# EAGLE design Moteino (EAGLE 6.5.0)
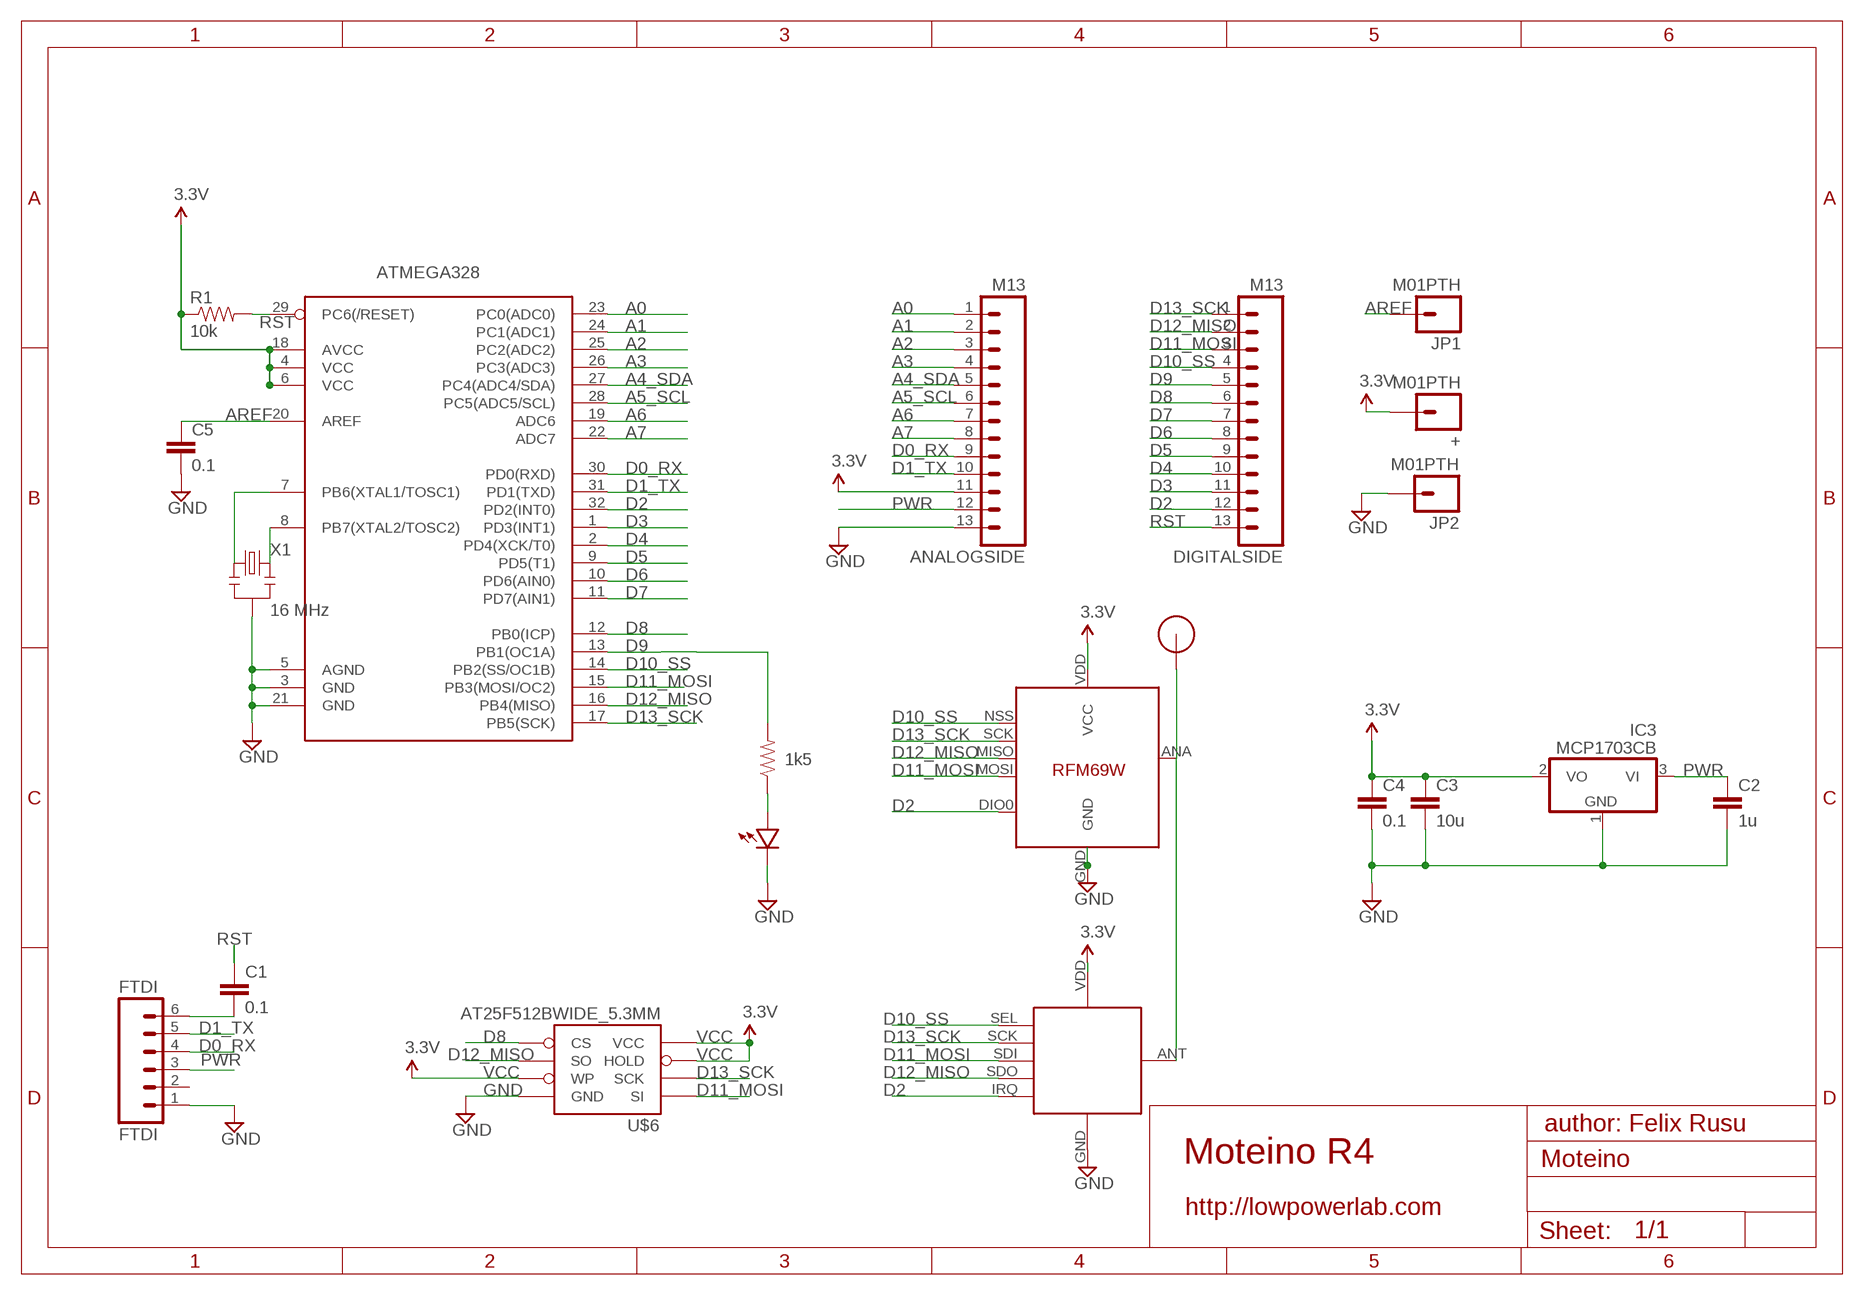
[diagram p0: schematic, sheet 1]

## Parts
+  M01PTH  [1X01]
ANALOGSIDE  M13  [1X13]
ATMEGA328  ATMega-328  ATMEGA168/328TQFP32  [TQFP32-08]
C1  0.1  CAP0603-CAP  [0603-CAP]
C2  1u  CAP0603-CAP  [0603-CAP]
C3  10u  CAP0805-CAP  [0805-CAP]
C4  0.1  CAP0603-CAP  [0603-CAP]
C5  0.1  CAP0603-CAP  [0603-CAP]
DIGITALSIDE  M13  [1X13]
FTDI  FTDI  M06SIP  [1X06]
IC3  MCP1703CB  [SOT23]
JP1  M01PTH  [1X01]
JP2  M01PTH  [1X01]
R1  10k  RESISTOR0603-RES  [0603-RES]
R2  1k5  RESISTOR0603-RES  [0603-RES]
RFM12B  RFM12B_MINPADS  [RFM12B-MINPADS]
U$1  RFM12B_ANTENNA  [RFM12B-ANTENNA]
U$2  LED0603  [0603-LED]
U$5  RFM69  [RFM69W-MINPADS]
U$6  AT25F512BWIDE_5.3MM  [SO08WIDE]
X1  16 MHz  RESONATORSMD  [RESONATOR-SMD]

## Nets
A0: ANALOGSIDE.1 ATMEGA328.23(PC0(ADC0))
A1: ANALOGSIDE.2 ATMEGA328.24(PC1(ADC1))
A2: ANALOGSIDE.3 ATMEGA328.25(PC2(ADC2))
A3: ANALOGSIDE.4 ATMEGA328.26(PC3(ADC3))
A4_SDA: ANALOGSIDE.5 ATMEGA328.27(PC4(ADC4/SDA))
A5_SCL: ANALOGSIDE.6 ATMEGA328.28(PC5(ADC5/SCL))
A6: ANALOGSIDE.7 ATMEGA328.19(ADC6)
A7: ANALOGSIDE.8 ATMEGA328.22(ADC7)
AREF: ATMEGA328.20(AREF) C5.1 JP1.1
D0_RX: ANALOGSIDE.9 ATMEGA328.30(PD0(RXD)) FTDI.4
D1_TX: ANALOGSIDE.10 ATMEGA328.31(PD1(TXD)) FTDI.5
D2: ATMEGA328.32(PD2(INT0)) DIGITALSIDE.12 RFM12B.IRQ U$5.DIO0
D3: ATMEGA328.1(PD3(INT1)) DIGITALSIDE.11
D4: ATMEGA328.2(PD4(XCK/T0)) DIGITALSIDE.10
D5: ATMEGA328.9(PD5(T1)) DIGITALSIDE.9
D6: ATMEGA328.10(PD6(AIN0)) DIGITALSIDE.8
D7: ATMEGA328.11(PD7(AIN1)) DIGITALSIDE.7
D8: ATMEGA328.12(PB0(ICP)) DIGITALSIDE.6 U$6.1(CS)
D9: ATMEGA328.13(PB1(OC1A)) DIGITALSIDE.5 R2.2
D10_SS: ATMEGA328.14(PB2(SS/OC1B)) DIGITALSIDE.4 RFM12B.SEL U$5.NSS(SEL)
D11_MOSI: ATMEGA328.15(PB3(MOSI/OC2)) DIGITALSIDE.3 RFM12B.SDI(SDI/MOSI) U$5.MOSI U$6.5(SI)
D12_MISO: ATMEGA328.16(PB4(MISO)) DIGITALSIDE.2 RFM12B.SDO(SDO/MISO) U$5.MISO U$6.2(SO)
D13_SCK: ATMEGA328.17(PB5(SCK)) DIGITALSIDE.1 RFM12B.SCK U$5.SCK U$6.6(SCK)
GND [power]: ANALOGSIDE.13 ATMEGA328.3(GND) ATMEGA328.5(AGND) ATMEGA328.21(GND) C2.2 C3.2 C4.2 C5.2 FTDI.1 IC3.1(GND) JP2.1 RFM12B.GND U$2.MINUS U$5.GND U$6.4(GND) X1.2
N$1: ATMEGA328.7(PB6(XTAL1/TOSC1)) X1.1
N$2: R2.1 U$2.PLUS
N$3: RFM12B.ANT U$1.P$1 U$5.ANA(ANT)
N$20: C1.2 FTDI.6
N$21: ATMEGA328.8(PB7(XTAL2/TOSC2)) X1.3
PWR [power]: ANALOGSIDE.12 C2.1 FTDI.3 IC3.3(VI)
RST: ATMEGA328.29(PC6(/RESET)) C1.1 DIGITALSIDE.13 R1.2
VCC: +.1 ANALOGSIDE.11 ATMEGA328.4(VCC) ATMEGA328.6(VCC) ATMEGA328.18(AVCC) C3.1 C4.1 IC3.2(VO) R1.1 RFM12B.VDD U$5.VDD(VCC) U$6.3(WP) U$6.7(HOLD) U$6.8(VCC) ; supply symbol labelled 3.3V
Unconnected: FTDI.2

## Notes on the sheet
- author: Felix Rusu
- Moteino R4
- http://lowpowerlab.com

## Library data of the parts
+ JP1 JP2 = SparkFun-Connectors:M01: Header 1
ANALOGSIDE DIGITALSIDE = SparkFun-Connectors:M13: 13-pin single row .1" header
ATMEGA328 = LowPowerLab:ATMEGA168/328: Atmel 32-pin 8-bit micro, 16k flash.
C1-C5 = LowPowerLab:CAP: Capacitor
FTDI = SparkFun-Connectors:M06: Header 6 Standard 6-pin 0.1" header. Use with straight break away headers (SKU : PRT-00116), right angle break away headers (PRT-00553), swiss pins (PRT-00743), machine pins (PRT-00117), and female headers (PRT-00115). Molex polarized connector foot print use with SKU : PRT-08094 with associated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
IC3 = linear:MCP1703: 250 mA, 16V, Low Quiescent Current LDO Regulator Source: http://ww1.microchip.com/downloads/en/DeviceDoc/22049b.pdf
R1 R2 = LowPowerLab:RESISTOR: Resistor
RFM12B = LowPowerLab:RFM12B_MINPADS
U$1 = LowPowerLab:RFM12B_ANTENNA
U$2 = LowPowerLab:LED
U$5 = LowPowerLab:RFM69
U$6 = LowPowerLab:AT25F512B: 4-Mbit SPI flash memory
X1 = SparkFun:RESONATOR: Resonator Small SMD resonator. This is the itty bitty 10/20MHz resonators with built in caps. CSTCE10M0G55 and CSTCE20M0V53. Footprint has been reviewed closely but hasn't been tested yet.

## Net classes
1 power: width 0.381 mm, clearance 0.254 mm

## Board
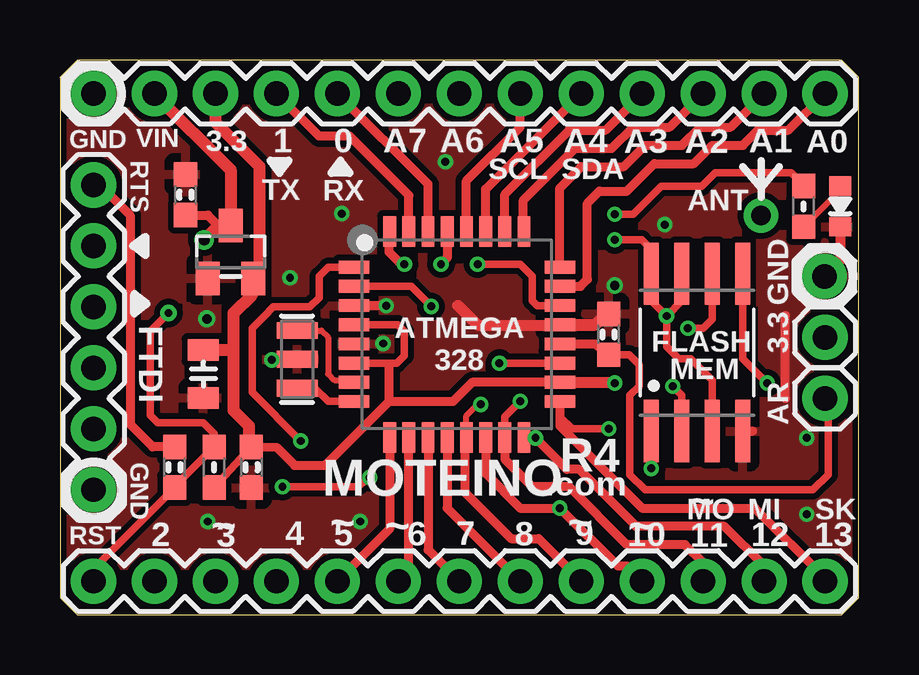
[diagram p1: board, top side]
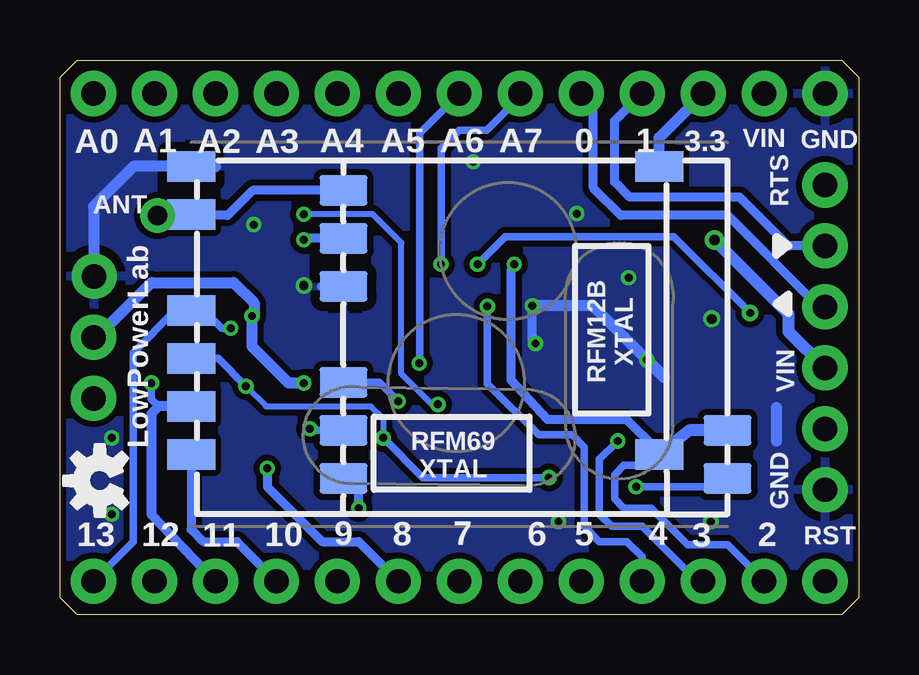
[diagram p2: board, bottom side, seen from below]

Size 33.27 x 23.11 mm. Coordinates in mm from the lower left corner, seen from the top.
Outline: 0.71,0 32.56,0 33.27,0.71 33.27,22.4 32.56,23.11 0.71,23.11 0,22.4 0,0.71 0.71,0
Copper layers (1*16): Top 0.035mm / dielectric 1.5mm / Bottom 0.035mm
Design rules "ITEADstudio_DRC *": minimum track width 6mil, minimum drill 12mil, track to track 6mil, track to pad 6mil, pad to pad 6mil, via to via 6mil, smd to smd 0mil, copper to edge 10mil, drill to drill 10mil, minimum pad ring 10mil, minimum via ring 6mil, stop-mask expansion 2mil, vias tented up to drill 100mil, thermal gap 15mil
tRestrict: area 24.3,8.9 to 29.1,12.8; area 5.8,16.9 to 6.9,18.5; area 5.2,9.7 to 6.7,10.4
bRestrict: area 27.4,17.7 to 29.2,18.7; area 21.1,13.8 to 22.9,14.9; area 21.6,12.6 to 22.1,13.2; area 20.7,12.6 to 21.2,13.2; area 20.2,12.8 to 20.7,13.5; area 20.1,13.4 to 20.6,14; area 26.5,18.9 to 27.1,19.5; area 26.5,17.9 to 27.1,18.5; area 27.5,19.1 to 28,19.8; area 27.9,18.8 to 29.1,19.6

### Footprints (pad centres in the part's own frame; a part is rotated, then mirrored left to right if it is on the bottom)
1X01 = drill 1.016 pad 1.88: 1 0,0
1X13 = drill 1.016 pad 1.88: 1 0,0; 2 2.54,0; 3 5.08,0; 4 7.62,0; 5 10.16,0; 6 12.7,0; 7 15.24,0; 8 17.78,0; 9 20.32,0; 10 22.86,0; 11 25.4,0; 12 27.94,0; 13 30.48,0
TQFP32-08 = smd 1.27 x 0.533: 1 -4.293,2.8; 2 -4.293,2; 3 -4.293,1.2; 4 -4.293,0.4; 5 -4.293,-0.4; 6 -4.293,-1.2; 7 -4.293,-2; 8 -4.293,-2.8; 17 4.293,-2.8; 18 4.293,-2; 19 4.293,-1.2; 20 4.293,-0.4; 21 4.293,0.4; 22 4.293,1.2; 23 4.293,2; 24 4.293,2.8 | smd 0.533 x 1.27: 9 -2.8,-4.293; 10 -2,-4.293; 11 -1.2,-4.293; 12 -0.4,-4.293; 13 0.4,-4.293; 14 1.2,-4.293; 15 2,-4.293; 16 2.8,-4.293; 25 2.8,4.293; 26 2,4.293; 27 1.2,4.293; 28 0.4,4.293; 29 -0.4,4.293; 30 -1.2,4.293; 31 -2,4.293; 32 -2.8,4.293
0603-CAP = smd 1.016 x 0.965: 1 -0.85,0; 2 0.85,0
0805-CAP = smd 0.902 x 1.3: 1 -1,0; 2 1,0
1X06 = drill 1.016 pad 1.88: 1 0,0; 2 2.54,0; 3 5.08,0; 4 7.62,0; 5 10.16,0; 6 12.7,0
SOT23 = smd 1 x 1.4: 1 -0.95,-1.1; 2 0.95,-1.1; 3 0,1.1
0603-RES = smd 1.016 x 0.965: 1 -0.85,0; 2 0.85,0
RFM12B-MINPADS = smd 2 x 1.27: ANT 8,-6; GND 8,-2; IRQ -8,4; SCK 8,4; SDI 8,2; SDO -8,6; SEL 8,6; VDD 8,-4
RFM12B-ANTENNA = drill 0.8 pad 1.422: P$1 0,0
0603-LED = smd 0.8 x 0.9: MINUS -0.85,0; PLUS 0.85,0
RFM69W-MINPADS = smd 2 x 1.27: ANA 8,-5; DIO0 -11.5,5; GND 8,-7; MISO 8,1; MOSI 8,3; NSS 8,5; SCK 8,-1; VDD -11.5,-7
SO08WIDE = smd 0.61 x 2.6: 1 -1.905,-3.269; 2 -0.635,-3.269; 3 0.635,-3.269; 4 1.905,-3.269; 5 1.905,3.286; 6 0.635,3.286; 7 -0.635,3.286; 8 -1.905,3.286
RESONATOR-SMD = smd 0.7 x 1.7: 1 -1.2,0; 2 0,0; 3 1.2,0

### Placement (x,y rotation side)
+  31.88,11.56 270 top
ANALOGSIDE  31.88,21.72 180 top
ATMEGA328  16.54,11.68 0 top
C1  4.78,6.15 90 top
C2  5.23,17.5 90 top
C3  5.97,10.03 270 top
C4  7.98,6.15 270 top
C5  22.86,11.68 90 top
DIGITALSIDE  31.88,1.4 180 top
FTDI  1.4,5.21 90 top
IC3  7.11,15.11 0 top
JP1  31.88,9.02 0 top
JP2  31.85,14.1 0 top
R1  6.43,6.15 90 top
R2  30.99,17.02 90 top
RFM12B  13.46,11.68 180 bottom
U$1  29.21,16.64 0 top
U$2  32.51,17.02 90 top
U$3  [OSHW-LOGO-S]  31.62,5.59 90 bottom
U$5  19.81,11.68 180 bottom
U$6  26.54,10.92 0 top
X1  9.88,10.64 270 top

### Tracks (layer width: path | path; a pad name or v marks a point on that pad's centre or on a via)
A0
  Top 0.381: ATMEGA328.23 21.68,13.68 21.97,13.97 21.97,17.14 22.48,17.65 23.62,17.65 24.77,18.8 26.42,18.8 27.18,19.56 28.45,19.56 29.08,20.19 30.35,20.19 ANALOGSIDE.1
A1
  Top 0.381: ATMEGA328.24 20.83,17.78 21.72,18.67 23.5,18.67 24.38,19.56 25.91,19.56 26.67,20.32 27.94,20.32 ANALOGSIDE.2
A2
  Top 0.381: ATMEGA328.25 19.3,15.98 19.3,17.27 21.46,19.43 22.99,19.43 23.88,20.32 25.4,20.32 ANALOGSIDE.3
A3
  Top 0.381: ATMEGA328.26 18.54,17.52 21.21,20.19 22.73,20.19 ANALOGSIDE.4
A4_SDA
  Top 0.381: ATMEGA328.27 17.73,17.73 ANALOGSIDE.5
A5_SCL
  Top 0.381: ATMEGA328.28 16.93,18.08 19.18,20.32 ANALOGSIDE.6
A6  (via drill 0.33)
  Top 0.305: ATMEGA328.19 v18.31,10.48
  Bottom 0.305: 18.29,10.41 18.29,20.07 ANALOGSIDE.7
  Bottom 0.381: 18.29,10.41 v18.31,10.48
A7  (via drill 0.33)
  Top 0.305: ATMEGA328.22 19.88,12.88 19.68,13.08 19.68,14.1 19.18,14.61 v17.4,14.61
  Bottom 0.305: v17.4,14.61 17.4,19.43 16.64,20.19 15.49,20.19 14.1,21.59 ANALOGSIDE.8
AREF
  Top 0.305: C5.1 23.71,10.83 24.13,10.41 24.13,9.53 23.75,9.14 23.75,5.84 24.38,5.21 31.37,5.21 32,5.84 32,8.89 JP1.1
  Top 0.381: ATMEGA328.20 22.28,11.28 C5.1
D0_RX
  Top 0.381: ATMEGA328.30 15.34,17.94 ANALOGSIDE.9
  Bottom 0.381: FTDI.4 1.65,12.83 5.46,16.64 9.91,16.64 11.05,17.78 11.05,21.21 ANALOGSIDE.9 11.68,21.59
D1_TX
  Top 0.381: ATMEGA328.31 14.54,17.47 12.06,19.94 10.79,19.94 ANALOGSIDE.10
  Bottom 0.381: FTDI.5 2.92,15.37 4.95,17.4 9.53,17.4 10.16,18.03 10.16,20.57 ANALOGSIDE.10
D2  (via drill 0.33)
  Top 0.381: v14.35,14.61 14.22,14.61 13.72,15.11 13.72,15.83 ATMEGA328.32
  Bottom 0.305: DIGITALSIDE.12 5.46,2.92 7.11,2.92 8.64,4.45 9.78,4.45 10.16,4.83 10.16,5.84 9.78,6.22 8.77,6.22 U$5.DIO0
  Bottom 0.381: 7.85,6.89 8.41,6.89 9.65,8.13 12.95,8.13 14.48,9.78 14.48,14.35 v14.35,14.61
  Bottom 0.406: U$5.DIO0 8.05,6.68 7.85,6.89
  Bottom 0.508: RFM12B.IRQ 7.06,7.68 U$5.DIO0
D3  (via drill 0.33)
  Top 0.305: v10.03,7.24 8,9.27 8,11.05 8,11.94 8.51,12.45 8.89,12.83 10.41,12.83 10.79,13.21 10.79,14.1 11.18,14.48 ATMEGA328.1
  Top 0.381: ATMEGA328.1
  Bottom 0.305: DIGITALSIDE.11 6.73,1.4 9.02,3.68 10.29,3.68 10.79,4.19 10.79,6.48 v10.03,7.24
D4  (via drill 0.33)
  Top 0.305: ATMEGA328.2 14.63,13.68 v15.46,12.85
  Top 0.381: 12.17,13.73 ATMEGA328.2
  Bottom 0.305: DIGITALSIDE.10 9.02,2.41 9.65,3.05 10.79,3.05 11.43,3.68 11.43,6.99 11.94,7.49 13.34,7.49 15.46,9.62 v15.46,12.85
D5
  Top 0.381: ATMEGA328.9 13.73,3.58 DIGITALSIDE.9
D6
  Top 0.381: DIGITALSIDE.8 14.54,1.83 ATMEGA328.10
D7
  Top 0.381: ATMEGA328.11 15.34,2.7 DIGITALSIDE.7
D8  (via drill 0.33)
  Top 0.305: v24.64,6.1 24.62,7.75 U$6.1
  Top 0.381: ATMEGA328.12 16.14,4.44 DIGITALSIDE.6
  Bottom 0.381: v24.64,6.1 24.64,5.33 22.35,3.05 20.83,3.05 DIGITALSIDE.6
D9  (via drill 0.33)
  Top 0.254: ATMEGA328.13 16.93,8.3 17.4,8.76 v17.53,8.76
  Top 0.305: R2.2 30.77,18.12 30.48,18.41 27.3,18.41 26.75,17.86 25.04,17.86 23.88,16.69 v23.11,16.69
  Top 0.381: ATMEGA328.13 16.89,7.31 16.89,5.08 18.8,3.17 19.94,3.17 DIGITALSIDE.5
  Bottom 0.254: v17.53,8.76 17.78,8.76 19.05,10.03 19.05,15.49 20.24,16.69 v23.11,16.69
D10_SS  (via drill 0.33)
  Top 0.381: ATMEGA328.14 17.73,5.89 19.18,4.45 v20.83,4.45 23.24,2.03 23.62,2.03 DIGITALSIDE.4
  Bottom 0.254: 20.83,5.43 RFM12B.SEL
  Bottom 0.381: v20.83,4.45 20.83,5.43 | U$5.NSS 27.81,3.56 27.3,3.05 25.91,3.05 DIGITALSIDE.4
D11_MOSI  (via drill 0.33)
  Top 0.305: v29.46,9.65 28.45,10.67 U$6.5 | ATMEGA328.15 18.54,8.25 v19.18,8.89
  Top 0.381: ATMEGA328.15 18.54,6.48 19.68,5.33 21.21,5.33 23.62,2.92 26.04,2.92 26.8,2.16 DIGITALSIDE.3
  Bottom 0.305: v29.46,9.65 29.46,8.99 29.16,8.68 | v19.18,8.89 19.97,9.68 RFM12B.SDI
  Bottom 0.381: DIGITALSIDE.3 29.46,4.19
  Bottom 0.406: U$5.MOSI 29.16,8.68 29.46,8.38 29.46,4.19
D12_MISO  (via drill 0.33)
  Top 0.305: v25.53,9.53 25.91,9.14 25.91,8.51 U$6.2 | v9.27,5.33 12.39,5.33 v12.9,5.71
  Top 0.381: ATMEGA328.16 19.91,7.39 v19.81,7.37 21.12,6.06 21.63,6.06 24,3.68 27.69,3.68 29.34,2.03 DIGITALSIDE.2
  Bottom 0.254: v25.53,9.53 24.69,8.69 20.32,8.69 19.81,8.18 v19.81,7.37
  Bottom 0.305: U$5.MISO 26.69,10.68 v25.53,9.53 25.84,9.84 | v19.81,7.37 18.16,5.71 v12.9,5.71 | v9.27,5.33 5.81,5.33 RFM12B.SDO
D13_SCK  (via drill 0.33)
  Top 0.305: v26.16,11.94 26.8,11.94 27.18,12.32 U$6.6 | v22.86,7.75 21.34,7.75 20.83,8.26
  Top 0.381: DIGITALSIDE.1 31.88,1.52 28.96,4.45 24.25,4.45 20.83,7.87 20.83,8.26 ATMEGA328.17
  Bottom 0.305: RFM12B.SCK 22.8,7.68 v22.86,7.75 | DIGITALSIDE.1 30.23,3.05 30.23,10.92 28.46,12.68 U$5.SCK 27.8,12.7 27.3,12.7 26.54,11.94 v26.16,11.94
GND  (via drill 0.33, 0.38, 0.41)
  Top 0.381: 20.94,12.06 ATMEGA328.21 | v13.59,12.88 ATMEGA328.3 | 16.53,12.88 16.59,12.88 | U$6.4 28.86,7.65 | 30.23,9.02 30.23,12.47 | v8.82,10.62 X1.2
  Top 0.406: U$2.MINUS 32.51,14.76 JP2.1
  Top 0.457: 20.94,12.06 17.4,12.06 16.59,12.88
  Top 0.508: ATMEGA328.21 22.28,12.08 C5.2 22.99,12.41
  Bottom 0.381: 13.59,12.81 v13.59,12.88 13.59,11.3 v13.46,11.3 | RFM12B.GND 22.38,13.68
  Bottom 0.457: 31.88,14.12 JP2.1 31.88,14.12 | 26.81,18.68 30.21,18.68 31.88,17.02 31.88,14.12 | v8.82,10.62 11.08,12.88 v13.59,12.88 | 3.43,8.64 3.43,7.24
  Bottom 0.508: U$5.GND 26.81,18.68 | 8.11,9.91 v8.82,10.62
  other vias: 6.12,12.32 23.11,13.72 6.15,3.89 12.5,3.89 9.58,14.05 11.74,16.71 16.06,18.87 25.2,16.26 31.11,7.37 31.11,4.19
  pour Bottom: -0.64,24 -0.64,-0.76 34.04,-0.76 34.04,24
  pour Top: -0.64,24 -0.64,-0.76 34.04,-0.76 34.04,24
N$1
  Top 0.254: X1.1 10.89,11.84 11.18,11.56 11.18,10.03 11.43,9.78 12.15,9.78 ATMEGA328.7
N$2
  Top 0.254: R2.1 32.38,17.57 U$2.PLUS
N$3
  Bottom 0.381: U$1.P$1 28.5,16.68 U$5.ANA 27.51,16.64 26.29,16.64 25.24,17.68 RFM12B.ANT
N$20
  Top 0.381: C1.2 3.86,7 2.92,7.94 2.92,16.64 1.65,17.91 FTDI.6
N$21
  Top 0.254: ATMEGA328.8
  Top 0.305: X1.3 10.62,9.44 11.18,8.89 ATMEGA328.8
PWR  (via drill 0.46 pad 0.81)
  Top 0.381: C2.1 6.17,16.65 6.6,16.21
  Top 0.508: ANALOGSIDE.12 7.11,18.54 IC3.3 6.6,16.21 v6,15.61
  Bottom 0.508: FTDI.3 2.92,11.81 2.92,12.45 2.92,12.53 v6,15.61
RST  (via drill 0.33, 0.33 pad 0.69)
  Top 0.305: DIGITALSIDE.13 1.4,1.92 C1.1 4.78,5.35 R1.2 6.43,7.54 5.97,8 4.06,8 3.76,8.31 3.76,11.81 v4.52,12.57
  Top 0.381: ATMEGA328.29 16.14,14.87 v15.88,14.61
  Bottom 0.305: v15.88,14.61 14.73,15.75 7.7,15.75 v4.52,12.57
VCC  (via drill 0.33)
  Top 0.305: ATMEGA328.4 14.08,12.08 14.35,11.81 14.35,10.79 14.03,10.48 13.84,10.48 | ATMEGA328.6 13.84,10.48 | v25.27,12.45 24.64,13.08 U$6.8 | v25.27,12.45 25.91,13.08 U$6.7 | v25.27,12.45 25.27,11.18 25.78,10.67 26.29,10.67 27.18,9.78 U$6.3 | v23.11,15.62 24.24,15.62 24.64,15.22 | 13.72,10.36 13.84,10.48 | R1.1 6.43,5.32 C4.1
  Top 0.381: 24.64,15.22 U$6.8 | ATMEGA328.18 17.18,9.68 16.38,8.89 13.72,8.89 | 13.72,8.89 13.72,10.36 | C4.1 9.03,6.97 9.78,6.22 11.05,6.22 13.72,8.89
  Top 0.457: ATMEGA328.18 23.21,9.68 v23.11,9.65
  Top 0.508: 7.87,7.07 C4.1 7.87,7.07 | C3.1 6.24,11.03 7.22,11.03 7.24,11.05 | 7.87,7.07 7.87,7.87 7.24,8.51 7.24,11.05 | 7.24,11.05 7.24,12.57 8,13.34 8,13.95 IC3.2 | IC3.2 8.23,13.84 | ANALOGSIDE.11 6.48,20.52 U$5.VDD 8.31,14.26 IC3.2
  Top 0.635: 8.23,13.73 8.23,13.84
  Bottom 0.381: RFM12B.VDD 23.18,15.68 v23.11,15.62
  Bottom 0.457: +.1 31.75,11.56 29.46,13.84 26.04,13.84 25.18,12.99 25.18,12.54 v25.27,12.45 25.27,11.18 23.75,9.65 v23.11,9.65 | U$5.VDD 8.31,19.88 ANALOGSIDE.11

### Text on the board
tPlace: R4 | MOTEINO | .com
bPlace: RFM12B / XTAL | LowPowerLab | RFM69 / XTAL
tDocu: REG
_tsilk: VIN | 3.3 | 1 | 0 | A7 | A6 | A5 | A4 | A3 | A2 | A1 | GND | RTS | A0 | TX | RX | SCL | SDA | ANT | GND | 3.3 | FLASH | ATMEGA / 328 | MEM | AR | FTDI | GND | 2 | 3 | 4 | 5 | 6 | 7 | 8 | 9 | 10 | MO | ~ | 11 | MI | 12 | SK | 13 | RST | ~ | ~ | ~ | ~ | ~
_bsilk: VIN | 3.3 | 1 | 0 | A7 | A6 | A5 | A4 | A3 | A2 | A1 | A0 | GND | RTS | ANT | VIN | GND | 2 | 3 | 4 | 5 | 6 | 7 | 8 | 9 | 10 | 11 | 12 | 13 | RST

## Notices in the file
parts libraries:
SparkFun-Connectors: Licensing: CC v3.0 Share-Alike You are welcome to use this library for commercial purposes.
